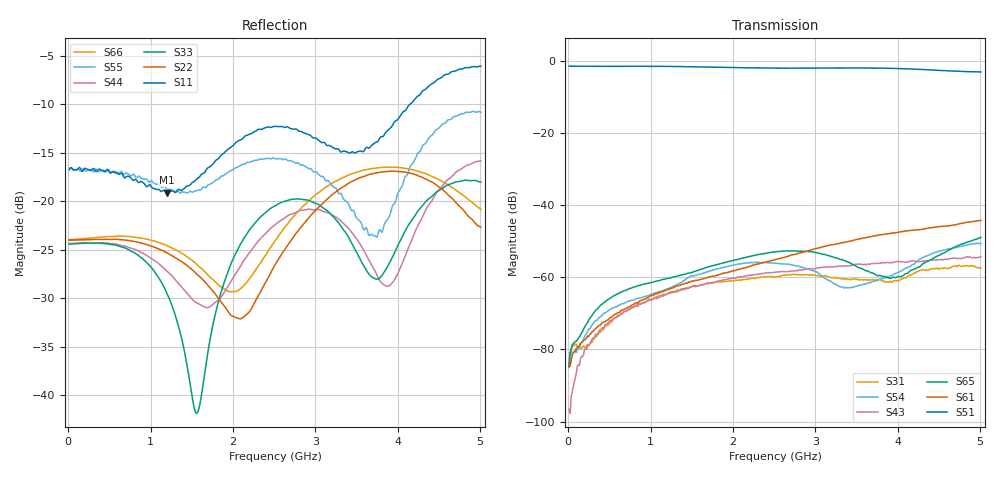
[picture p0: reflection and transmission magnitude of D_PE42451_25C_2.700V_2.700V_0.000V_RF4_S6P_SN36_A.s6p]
! Device ID: PE42451
! Serial: 36
! Insertion: A
! Temp: 25C
! VDD: 2.700
! Control_Hi: 100.000
! Control_Lo: 0.000
! Logic State: RF4
! Port 1: RFC
! Port 2: RF1
! Port 3: RF2
! Port 4: RF3
! Port 5: RF4
! Port 6: RF5
! V1 = 0.00
! V2 = 0.00
! V3 = 2.70
! V4 = 0.00
! IDD: 1.077020e-05
#  Hz  S  RI  R  50
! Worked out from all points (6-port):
!   401 points, 10 MHz to 5.01 GHz, reference 50 ohm
!   strongest paths, dB at 10 MHz, 1.26 GHz, 2.51 GHz, 3.76 GHz, 5.01 GHz:
!     S51: -1.5, -1.6, -2.1, -2.1, -3.1
!     S61: -84.2, -63.0, -55.1, -48.3, -44.3
!     S65: -84.8, -60.0, -53.0, -59.6, -49.0
!     S43: -96.6, -64.1, -58.7, -56.2, -54.3
!     S54: -85.0, -62.7, -56.1, -60.9, -50.7
!     S31: -83.8, -64.0, -59.9, -60.8, -57.5
!   lowest |S11| = -19.1 dB at 1.198 GHz (marker M1), VSWR 1.25, Z = 56.1 - j10.1 ohm
!   |S11| at or under -10 dB: start of sweep to 4.147 GHz
